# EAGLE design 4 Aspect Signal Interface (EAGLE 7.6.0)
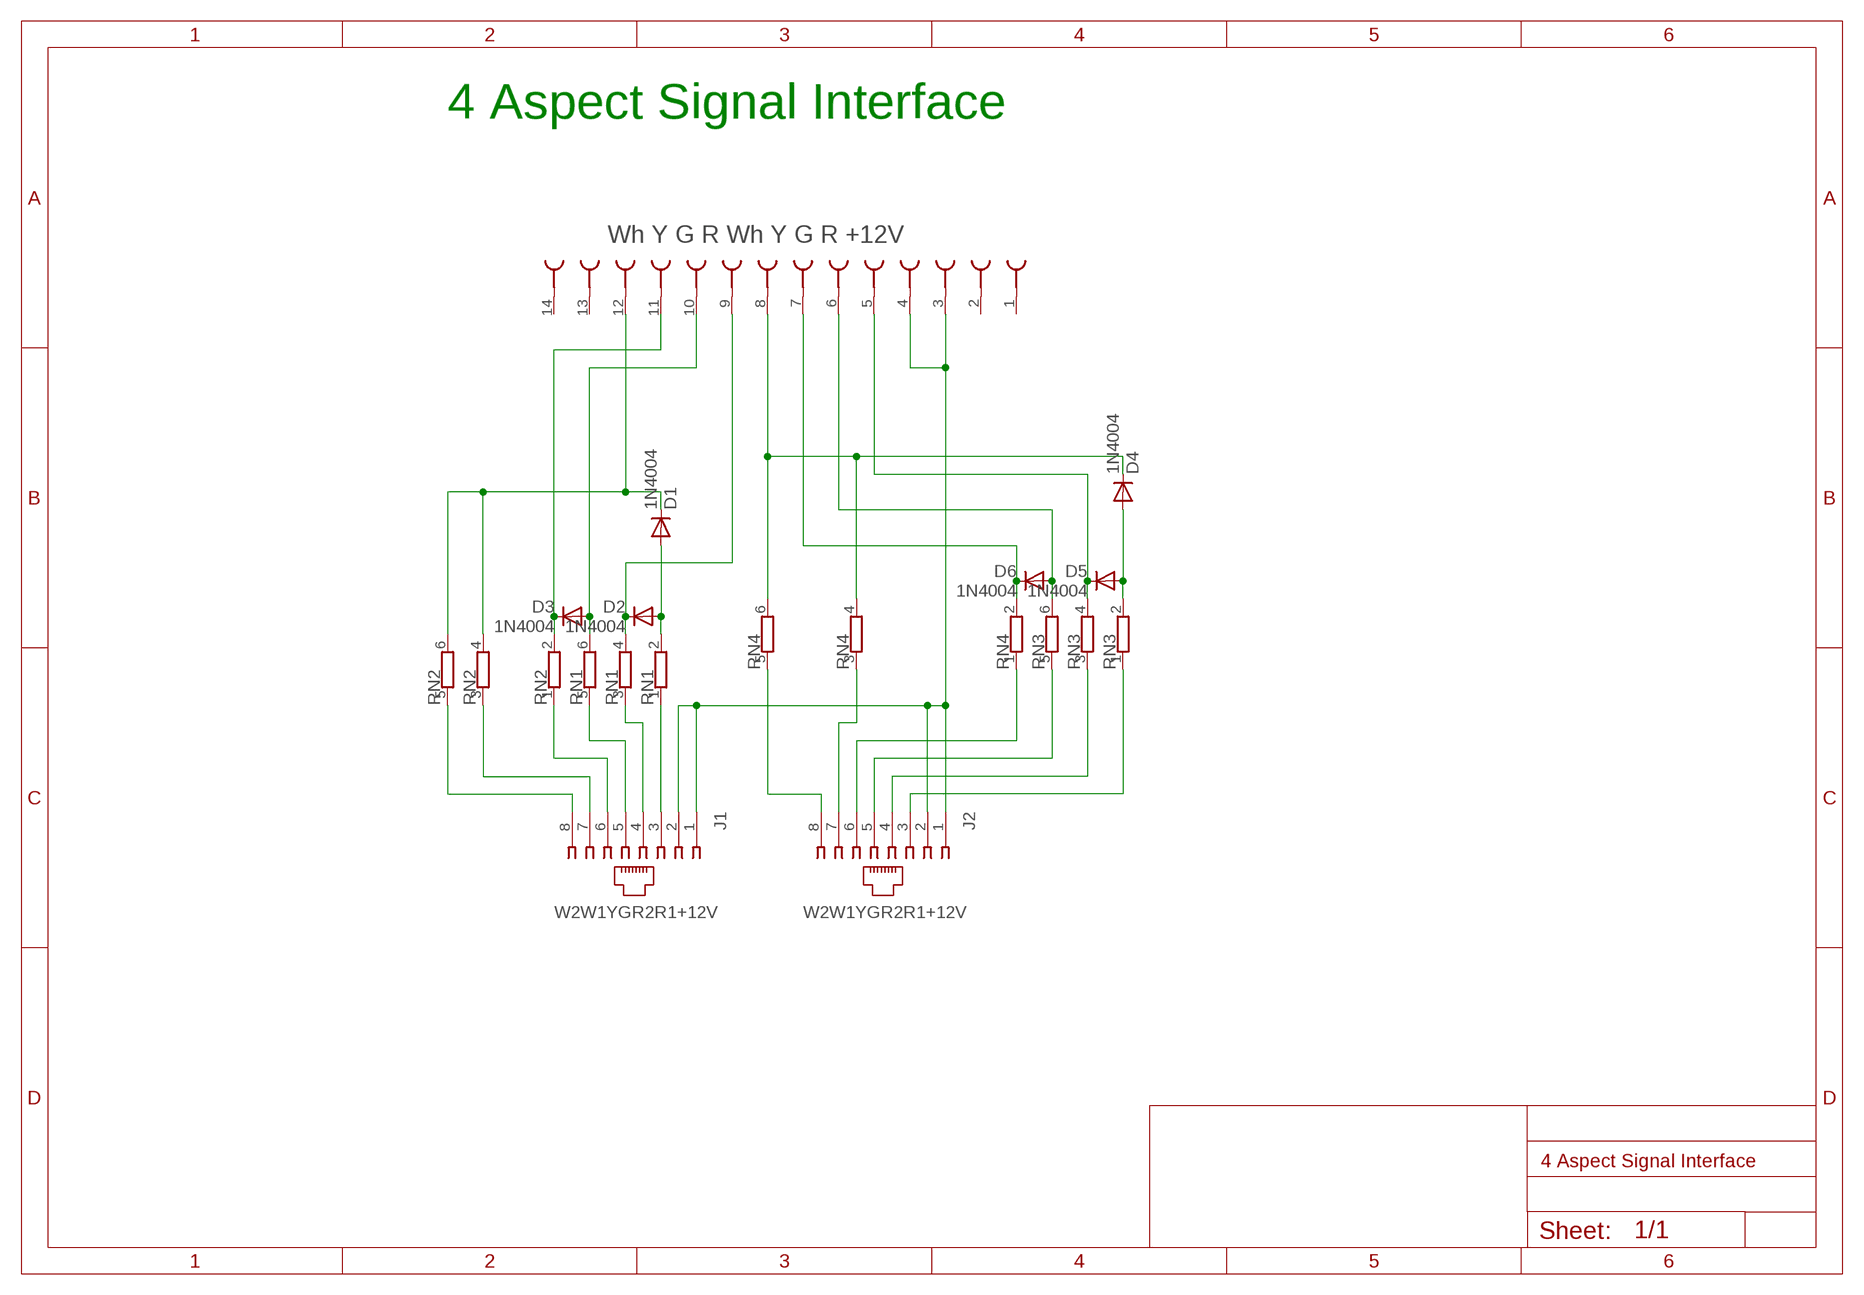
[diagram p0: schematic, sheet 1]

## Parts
D1  1N4004  [DO41-10]
D2  1N4004  [DO41-10]
D3  1N4004  [DO41-10]
D4  1N4004  [DO41-10]
D5  1N4004  [DO41-10]
D6  1N4004  [DO41-10]
J1  520251-4  [520251-4]
J2  520251-4  [520251-4]
RN1  E3RP  [SIL6]
RN2  E3RP  [SIL6]
RN3  E3RP  [SIL6]
RN4  E3RP  [SIL6]
U$1  AMP_FEMALE_PLUG  [AMP_FEMALE_PLUG]

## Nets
N$1: J1.1 J1.2 J2.1 J2.2 U$1.3(SK2) U$1.4(SK3)
N$2: J2.8 RN4.5
N$3: D2.C RN1.4 U$1.9(SK8)
N$4: D3.A RN1.6 U$1.10(SK9)
N$5: D3.C RN2.2 U$1.11(SK10)
N$6: D1.C RN2.4 RN2.6 U$1.12(SK11)
N$7: J1.3 RN1.1
N$8: J1.4 RN1.3
N$9: J1.5 RN1.5
N$10: J1.6 RN2.1
N$11: J1.7 RN2.3
N$12: J1.8 RN2.5
N$13: J2.7 RN4.3
N$14: D1.A D2.A RN1.2
N$15: D5.C RN3.4 U$1.5(SK4)
N$16: D6.A RN3.6 U$1.6(SK5)
N$17: D6.C RN4.2 U$1.7(SK6)
N$18: D4.C RN4.4 RN4.6 U$1.8(SK7)
N$19: J2.6 RN4.1
N$20: J2.5 RN3.5
N$21: J2.4 RN3.3
N$22: J2.3 RN3.1
N$25: D4.A D5.A RN3.2
Unconnected: U$1.1(SK) U$1.2(SK1) U$1.13(SK12) U$1.14(SK13)

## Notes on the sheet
- 4 Aspect Signal Interface
- Wh Y G R Wh Y G R +12V
- W2W1YGR2R1+12V | W2W1YGR2R1+12V

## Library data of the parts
D1-D6 = diode:1N4004: DIODE
J1 J2 = con-amp:520251-4: AMP connector; MF: TYCO ELECTRONICS; MPN: 5520251-4; OC_FARNELL: 1557070; OC_NEWARK: 42K7223
RN1-RN4 = resistor-sil:E3RP: SIL RESISTOR; OC_FARNELL: unknown; OC_NEWARK: unknown
U$1 = con-3m:AMP_FEMALE_PLUG

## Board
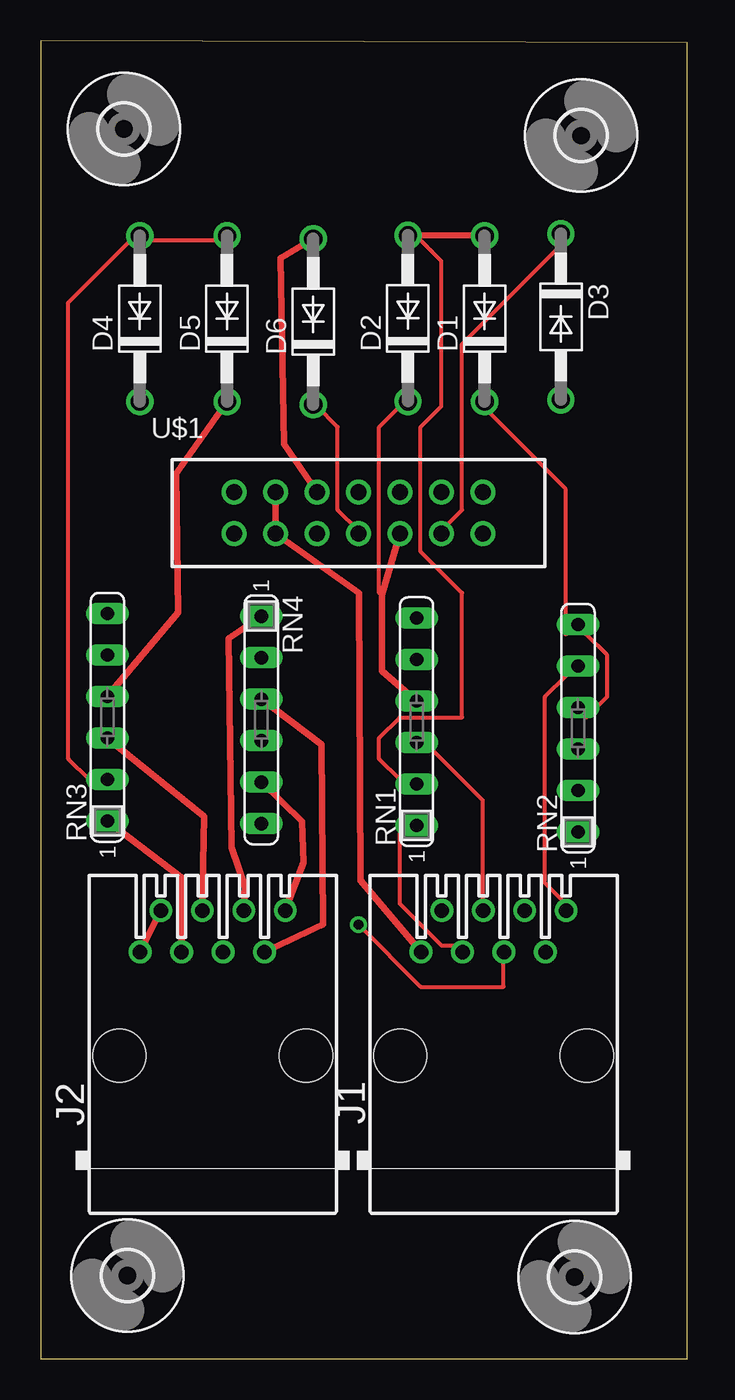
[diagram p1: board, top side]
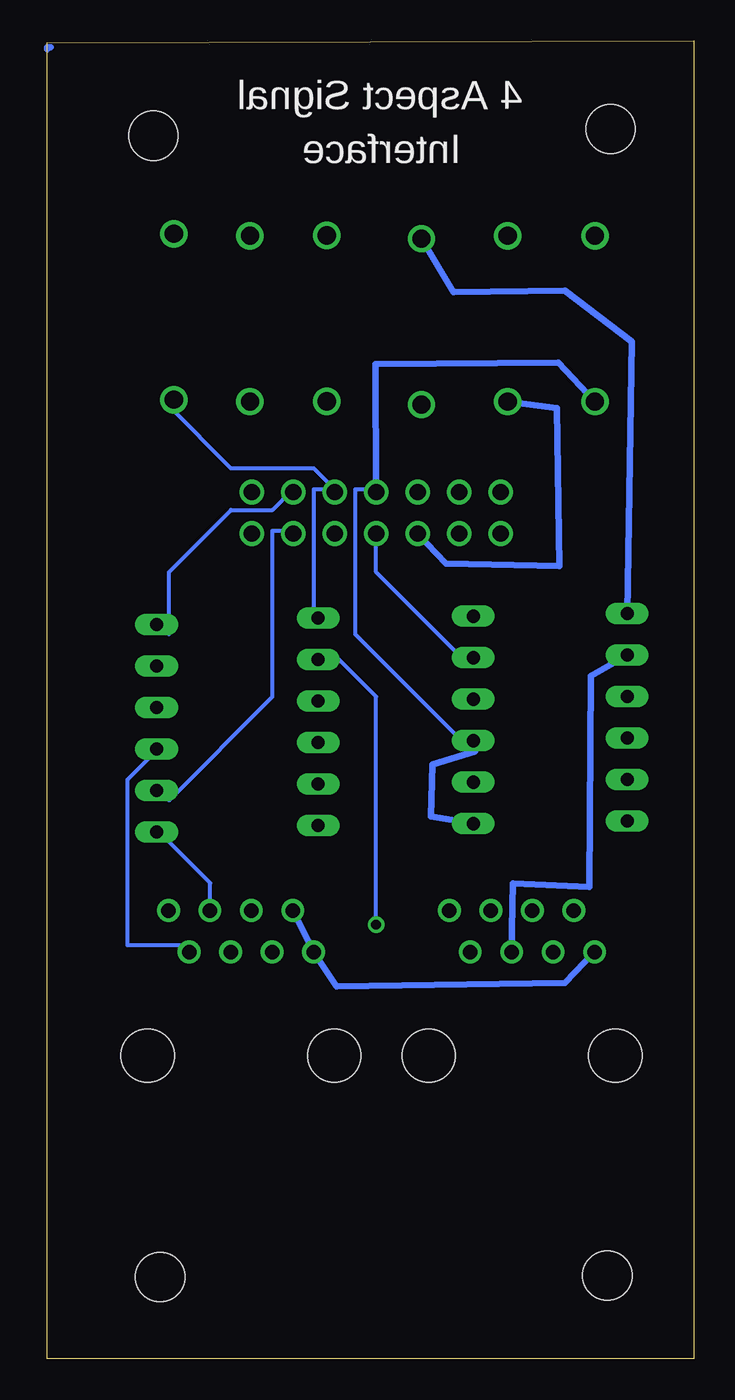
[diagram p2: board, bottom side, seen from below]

Size 39.6 x 80.7 mm. Coordinates in mm from the lower left corner, seen from the top.
Outline: 0,0 39.6,0 39.6,80.6 0,80.7 0,0
Copper layers (1*16): Top 0.035mm / dielectric 1.5mm / Bottom 0.035mm
Design rules "default": minimum track width 10mil, minimum drill 24mil, track to track 8mil, track to pad 8mil, pad to pad 8mil, via to via 8mil, smd to smd 8mil, copper to edge 40mil, drill to drill 8mil, minimum pad ring 10mil, minimum via ring 8mil, stop-mask expansion 4mil, vias tented up to drill 0mil, thermal gap 10mil

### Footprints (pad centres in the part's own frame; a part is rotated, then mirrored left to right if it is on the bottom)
DO41-10 = drill 1.118: A 5.08,0; C -5.08,0
520251-4 = drill 0.889: 1 -4.445,6.35; 2 -3.175,8.89; 3 -1.905,6.35; 4 -0.635,8.89; 5 0.635,6.35; 6 1.905,8.89; 7 3.175,6.35; 8 4.445,8.89 | hole 3.251: -5.715,0; 5.715,0
SIL6 = drill 0.813 long: 1 -6.35,0; 2 -3.81,0; 3 -1.27,0; 4 1.27,0; 5 3.81,0; 6 6.35,0
AMP_FEMALE_PLUG = drill 1 pad 1.422: 1 -10.16,-1.27; 2 -10.16,1.27; 3 -7.62,-1.27; 4 -7.62,1.27; 5 -5.08,-1.27; 6 -5.08,1.27; 7 -2.54,-1.27; 8 -2.54,1.27; 9 0,-1.27; 10 0,1.27; 11 2.54,-1.27; 12 2.54,1.27; 13 5.08,-1.27; 14 5.08,1.27
3,0 = hole 3: 0,0

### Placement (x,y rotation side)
D1  27.19,63.69 90 top
D2  22.49,63.71 90 top
D3  31.86,63.81 270 top
D4  6.06,63.69 90 top
D5  11.41,63.69 90 top
D6  16.69,63.51 90 top
J1  27.74,18.56 0 top
J2  10.53,18.56 0 top
RN1  23.02,39.01 90 top
RN2  32.91,38.61 90 top
RN3  4.08,39.28 90 top
RN4  13.51,39.12 270 top
U$1  22,51.8 0 top
U$3  [3,0]  5.3,5.1 0 top
U$4  [3,0]  32.7,5 0 top
U$6  [3,0]  5.1,75.3 0 top
U$17  [3,0]  33.1,74.9 0 top

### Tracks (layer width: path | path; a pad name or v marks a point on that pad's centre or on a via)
N$1
  Top 0.406: J2.1 J2.2 | J1.1 19.6,29.3 19.5,46.9 U$1.3 U$1.4
  Bottom 0.406: J2.1 7.9,23 21.9,22.8 J1.1 J1.2
N$2
  Top 0.406: J2.8 16.1,30.4 16,32.9 RN4.5
N$3
  Top 0.254: D2.C 22,58.33 20.73,57.06 20.73,46.9 20.9,46.8
  Top 0.406: U$1.9 20.9,46.8 20.9,42.1 RN1.4
N$4
  Bottom 0.254: 22,53.25 23.27,53.25 23.27,45.63 RN1.6 | 22,53.25 23.27,54.52 28.35,54.52 32.16,58.33 D3.A | 22,53.25 U$1.10
N$5
  Top 0.254: D3.C 32.16,68.49 25.81,62.14 25.81,51.98 24.54,50.71 U$1.11
  Bottom 0.254: RN2.2 32.16,34.2 25.81,40.55 25.81,50.71 24.54,50.71 U$1.11
N$6
  Top 0.254: RN2.4 33.43,39.28 34.7,40.55 34.7,43.09 33.43,44.36 RN2.6 32.16,44.36 32.16,53.25 27.08,58.33 D1.C
  Bottom 0.254: U$1.12 24.54,53.25 25.81,51.98 28.35,51.98 32.16,48.17 32.16,44.36 RN2.6
N$7
  Top 0.254: RN1.1 22,32.93 22,27.85 24.54,25.31 25.81,25.31 J1.3
  Top 0.406: J1.3 25.5,25
N$8
  Top 0.254: RN1.3 23.27,38.01 27.08,34.2 27.08,27.85 J1.4
N$9  (via drill 0.61)
  Top 0.254: v19.46,26.58 23.27,22.77 28.35,22.77 28.35,25.31 J1.5
  Bottom 0.254: v19.46,26.58 19.46,40.55 22,43.09 RN1.5
N$10
  Bottom 0.254: RN2.1 32.16,31.66 29.62,29.12 29.62,27.85 J1.6
N$11
  Bottom 0.254: RN2.3 33.43,36.74 34.7,35.47 34.7,25.31 30.89,25.31 J1.7
N$12
  Top 0.254: RN2.5 32.16,41.82 30.89,40.55 30.89,29.12 32.16,27.85 J1.8
N$13
  Top 0.406: RN4.3 13.4,40.5 17.2,37.6 17.3,26.6 J2.7
N$14
  Top 0.254: RN1.2 22,35.47 20.73,36.74 20.73,38.01 22,39.28 25.81,39.28 25.81,46.9 23.27,49.44 23.27,57.06 24.54,58.33 24.54,67.22 23.27,68.49 D2.A
  Top 0.406: D2.A D1.A
  Bottom 0.406: D1.A 26.8,68.7 26.7,68.7 26.8,68.8 27.2,68.7 | 27.2,68.7 27.2,68.8 | 27.2,68.7 27.1,68.8 27.2,68.8 | 27.2,68.8 27.3,68.8
N$15
  Top 0.406: RN3.4 8.4,45.7 8.3,54.2 D5.C
  Bottom 0.406: U$1.5 15.2,48.7 8.24,48.53 8.4,58.2 D5.C
N$16
  Top 0.406: D6.A 14.7,67.4 14.9,56 U$1.6
  Bottom 0.406: RN3.6 3.8,62.3 7.9,65.4 14.74,65.31 D6.A
N$17
  Top 0.254: D6.C 16.92,58.33 18.19,57.06 18.19,51.98 19.46,50.71 U$1.7
  Bottom 0.254: RN4.2 14.38,43.09 19.46,48.17 U$1.7 19.46,50.71
N$18
  Bottom 0.254: RN4.4 14.38,38.01 20.73,44.36 20.73,53.25 19.46,53.25 U$1.8
  Bottom 0.406: D4.C 8.3,61 19.5,60.9 U$1.8 | RN4.4 13.4,37.2 16,36.4 16.1,33.2 RN4.6
N$19
  Top 0.406: RN4.1 11.5,44.1 11.7,31.3 12.5,28.9 J2.6
N$20
  Bottom 0.406: RN3.5 6.3,41.8 6.4,28.9 11.1,29.1 J2.5
N$21
  Top 0.406: RN3.3 10,33.2 J2.4
N$22
  Top 0.406: RN3.1 8.7,29.4 J2.3
N$25
  Top 0.254: RN3.2 2.95,35.47 1.68,36.74 1.68,64.68 5.49,68.49 D4.A 6.76,68.49 11.84,68.49 D5.A
N$83
  Bottom 0.406: 39.4,80.3 39.6,80.3 39.6,80.2

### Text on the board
bPlace: 4 Aspect Signal | Interface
